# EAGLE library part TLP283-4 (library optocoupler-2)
TOSHIBA PHOTOCOUPLER GaAs IRED & PHOTO-TRANSISTOR Source: http://www.semicon.toshiba.co.jp/td/en/Opto/Photocoupler/en_20050928_TLP283_datasheet.pdf
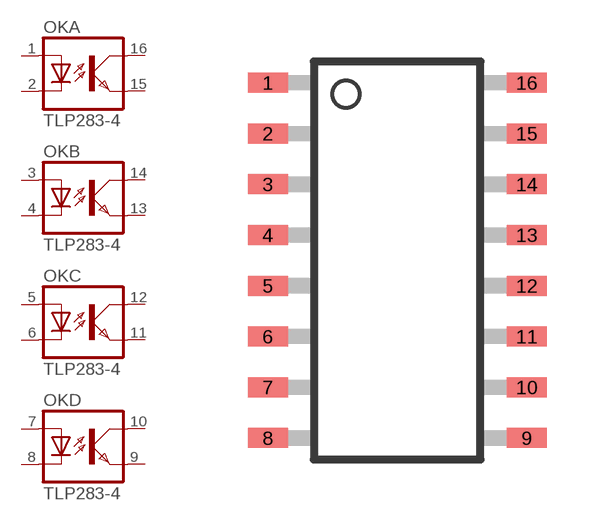
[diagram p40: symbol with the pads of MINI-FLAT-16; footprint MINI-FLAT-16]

Designator prefix OK; gates A=OK B=OK C=OK D=OK

## TLP283-4  [MINI-FLAT-16]
1  A:A  pas
2  A:C  pas
3  B:A  pas
4  B:C  pas
5  C:A  pas
6  C:C  pas
7  D:A  pas
8  D:C  pas
9  D:EMIT  pas
10  D:COL  pas
11  C:EMIT  pas
12  C:COL  pas
13  B:EMIT  pas
14  B:COL  pas
15  A:EMIT  pas
16  A:COL  pas

## Footprint MINI-FLAT-16 (pad centres in mm)
TOSHIBA PHOTOCOUPLER GaAs IRED & PHOTO-TRANSISTOR 11-10F1 Source: http://www.semicon.toshiba.co.jp/td/en/Opto/Photocoupler/en_20050928_TLP283_datasheet.pdf
smd 1 x 0.5: 1 -3.24,4.445; 2 -3.24,3.175; 3 -3.24,1.905; 4 -3.24,0.635; 5 -3.24,-0.635; 6 -3.24,-1.905; 7 -3.24,-3.175; 8 -3.24,-4.445; 9 3.24,-4.445; 10 3.24,-3.175; 11 3.24,-1.905; 12 3.24,-0.635; 13 3.24,0.635; 14 3.24,1.905; 15 3.24,3.175; 16 3.24,4.445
